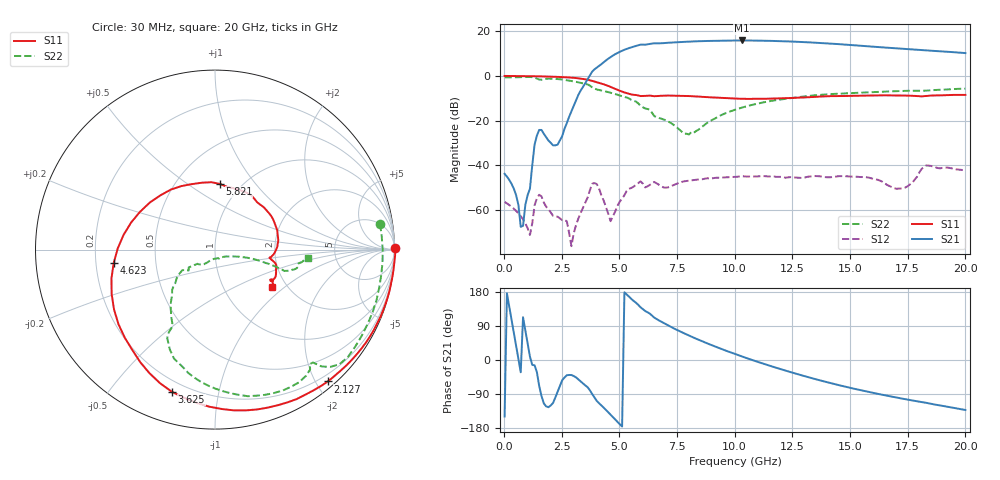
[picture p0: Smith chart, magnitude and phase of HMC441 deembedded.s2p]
!Hittite Microwave Corporation
!12 Elizabeth Drive
!Chelmsford, MA 01824
!Tel: 978-250-3343
!Fax: 978-250-3373
!Device: HMC441, 6-18 GHz GaAs PHEMT MMIc Medium Power Amplifier
!Misc: Vdd1 = Vdd2 = +5V, Vgg1 = vgg2 = Open, Room
# MHZ S MA R 50
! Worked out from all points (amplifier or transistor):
!   201 points, 30 MHz to 20 GHz, reference 50 ohm
!   highest |S21| = 15.9 dB at 10.31 GHz (marker M1)
!   |S21| within 3 dB of that: 5.548 GHz to 16.28 GHz (10.73 GHz wide, 98.3 % of centre)
!   unconditionally stable (mu >= 1): 523.3 MHz to end of sweep
!   at 3.325 GHz: K = 146.62, MAG = 2.7 dB, |S12| = -61.4 dB
!   at 10.02 GHz: K = 12.72, MAG = 16.5 dB, |S12| = -45.2 dB
!   at 20 GHz: K = 12.53, MAG = 12.3 dB, |S12| = -42.3 dB
!   S11 on the Smith chart (normalised r, x): 30 MHz: open; 2.127 GHz: 0.10, -2.17; 3.625 GHz: 0.15, -0.73; 4.623 GHz: 0.28, -0.06; 5.821 GHz: 0.80, +0.68; 20 GHz: 1.67, -0.81
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30  1.005 0.4  0.006442 -149.1  0.001517 123.2  0.931 8.8
828.8  0.997 -17.7  0.0004422 112.9  0.0006137 -99.8  0.946 -25.9
1128.35  0.993 -24.4  0.003009 8.8  0.0002753 176.7  0.952 -38.9
1427.9  0.988 -31.4  0.046 -31.8  0.001827 95.0  0.88 -47.7
2126.85  0.967 -49.4  0.028 -113.5  0.0007398 -36.0  0.871 -64.3
2925.65  0.921 -75.3  0.162 -39.6  0.0001542 -153.6  0.776 -89.6
3424.9  0.861 -96.6  0.567 -61.9  0.001118 33.8  0.684 -104.5
3624.6  0.828 -106.8  0.831 -71.7  0.001883 19.5  0.649 -110.6
4024  0.726 -129.1  1.545 -107.9  0.003805 -91.9  0.5 -119.0
4623.1  0.57 -172.3  2.66 -144.4  0.0005595 107.6  0.422 -125.6
5222.2  0.429 135.2  3.881 178.7  0.002146 -20.3  0.341 -134.5
5821.3  0.367 85.9  4.886 145.5  0.003994 -67.3  0.244 -145.5
6719.95  0.36 40.7  5.404 104.4  0.003659 -114.7  0.115 -133.8
8117.85  0.353 6.5  5.933 61.9  0.004574 -125.3  0.055 -66.1
9116.35  0.329 -4.0  6.169 36.4  0.005201 -140.3  0.11 -20.3
10015  0.312 -8.0  6.261 15.8  0.00551 -150.3  0.176 -14.6
10314.55  0.309 -8.3  6.267 9.2  0.005687 -152.3  0.196 -13.9
11512.75  0.31 -9.0  6.153 -15.1  0.005633 -161.5  0.273 -14.4
13409.9  0.339 -12.1  5.614 -49.0  0.00571 -162.3  0.368 -16.2
15007.5  0.359 -18.6  4.973 -73.7  0.005591 -164.4  0.413 -16.8
16704.95  0.369 -25.2  4.28 -95.4  0.003444 -164.0  0.453 -14.2
20000  0.378 -33.4  3.269 -131.9  0.007689 -140.2  0.522 -4.9
